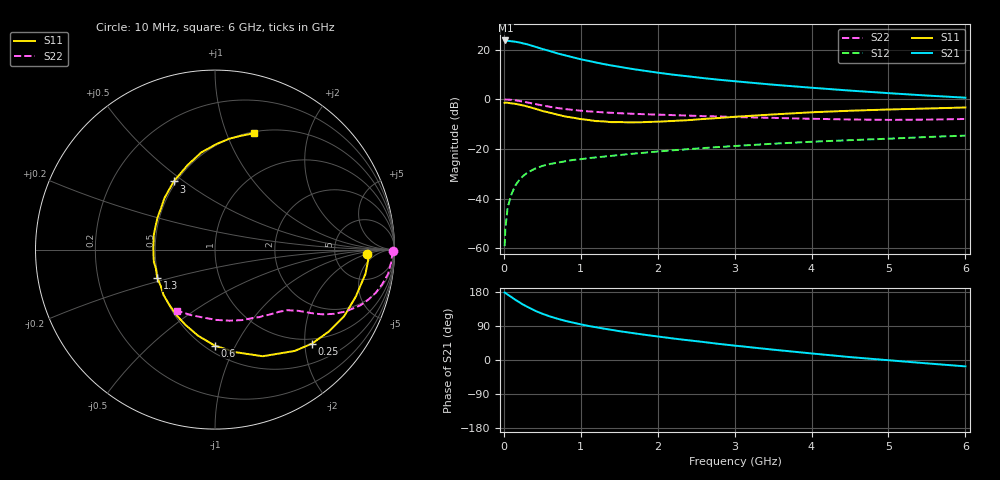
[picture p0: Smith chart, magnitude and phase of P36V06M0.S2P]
! SIEMENS Small Signal Semiconductors
! BFP181
! Si NPN RF Bipolar Junction Transistor in SOT143
! VCE = 6 V  IC = 6 mA
! Common Emitter S-Parameters:  March  1996
# GHz  S  MA  R  50
!  f  S11  S21  S12  S22
! GHz  MAG  ANG  MAG  ANG  MAG  ANG  MAG  ANG
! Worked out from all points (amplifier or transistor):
!   36 points, 10 MHz to 6 GHz, reference 50 ohm
!   highest |S21| = 23.7 dB at 20 MHz (marker M1)
!   |S21| within 3 dB of that: start of sweep to 456.1 MHz
!   unconditionally stable (mu >= 1): 1.658 GHz to end of sweep
!   at 250 MHz: K = 0.23, MSG = 26.7 dB, |S12| = -30.9 dB
!   at 1.4 GHz: K = 0.93, MSG = 18.2 dB, |S12| = -22.8 dB
!   at 6 GHz: K = 1.04, MAG = 6.4 dB, |S12| = -14.6 dB
!   S11 on the Smith chart (normalised r, x): 10 MHz: 12, -2; 250 MHz: 0.89, -2.16; 600 MHz: 0.55, -0.83; 1.3 GHz: 0.49, -0.18; 3 GHz: 0.48, +0.46; 6 GHz: 0.52, +1.26
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0.01  0.8488 -1.8  15.23 178.1  0.0011 87.3  0.9893 -0.6
0.02  0.8551 -4.0  15.3 177.1  0.0025 92.2  0.9878 -1.6
0.05  0.8496 -9.0  15.07 172.6  0.0067 87.2  0.9843 -4.1
0.15  0.8098 -27.2  14.42 158.9  0.0184 75.4  0.9506 -11.8
0.2  0.7812 -35.8  13.98 152.5  0.0236 72.0  0.9269 -15.1
0.25  0.7525 -44.1  13.37 146.2  0.0284 67.5  0.8967 -18.3
0.3  0.7183 -51.8  12.85 141.0  0.0328 63.6  0.8669 -21.0
0.4  0.6509 -65.9  11.54 130.6  0.0398 58.2  0.8064 -25.3
0.5  0.582 -78.9  10.31 122.1  0.0454 53.4  0.7524 -28.4
0.6  0.5347 -90.2  9.35 114.9  0.0498 50.7  0.7047 -30.8
0.7  0.4887 -101.2  8.369 108.8  0.0529 48.7  0.6655 -32.5
0.8  0.4505 -111.4  7.653 103.2  0.0565 46.8  0.6349 -33.7
1  0.3998 -129.4  6.392 94.1  0.0621 44.2  0.5888 -35.7
1.1  0.3825 -138.5  5.938 89.9  0.0653 43.5  0.5709 -36.6
1.3  0.3587 -154.0  5.112 82.8  0.0701 42.6  0.5445 -38.5
1.7  0.3438 178.0  4.012 70.3  0.0807 41.4  0.5093 -42.3
2.2  0.3663 151.2  3.133 56.8  0.0939 39.6  0.4794 -48.2
3  0.4439 121.2  2.311 38.0  0.1145 35.5  0.439 -59.7
3.5  0.4948 108.0  1.967 27.3  0.1273 32.5  0.422 -68.4
4.5  0.5877 89.3  1.496 7.7  0.1502 25.5  0.3919 -88.9
5.5  0.6517 76.9  1.189 -8.9  0.1738 19.5  0.3892 -110.7
6  0.6839 71.4  1.077 -16.8  0.1853 15.7  0.4006 -122.1
